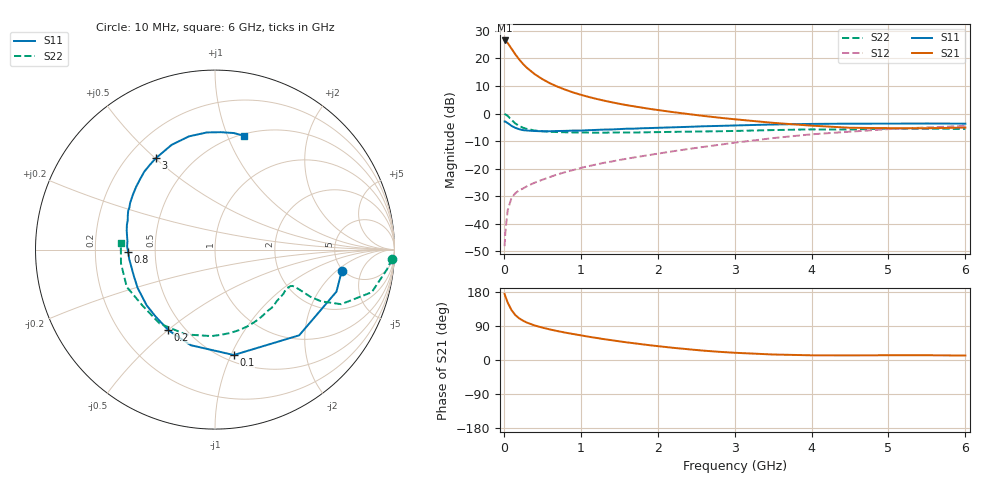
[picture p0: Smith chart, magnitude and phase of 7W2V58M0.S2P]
! Infineon Technologies  Discrete & RF Semiconductors
! BFS17W
! Si NPN RF Bipolar Junction Transistor in SOT323
! VCE = 2.5 V  IC = 8 mA
! Common Emitter S-Parameters:  August  1999
# GHz  S  MA  R  50
!  f  S11  S21  S12  S22
! GHz  MAG  ANG  MAG  ANG  MAG  ANG  MAG  ANG
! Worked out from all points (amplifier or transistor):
!   36 points, 10 MHz to 6 GHz, reference 50 ohm
!   highest |S21| = 26.5 dB at 10 MHz (marker M1)
!   |S21| within 3 dB of that: start of sweep to 100.4 MHz
!   unconditionally stable (mu >= 1): 434.1 MHz to 2.844 GHz; 4.192 GHz to end of sweep
!   at 250 MHz: K = 0.75, MSG = 22.6 dB, |S12| = -27.2 dB
!   at 1.4 GHz: K = 1.24, MAG = 7.8 dB, |S12| = -17.5 dB
!   at 6 GHz: K = 1.08, MAG = -2.0 dB, |S12| = -4.5 dB
!   S11 on the Smith chart (normalised r, x): 10 MHz: 4.84, -2.37; 100 MHz: 0.56, -1.02; 200 MHz: 0.41, -0.50; 800 MHz: 0.35, -0.01; 3 GHz: 0.31, +0.50; 6 GHz: 0.52, +1.15
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0.01  0.7161 -9.6  21.2 174.4  0.0039 85.6  0.9883 -2.9
0.02  0.7161 -19.1  20.9 168.0  0.007 81.2  0.9643 -6.6
0.05  0.6694 -45.5  19.09 151.5  0.0176 69.8  0.9052 -15.2
0.1  0.5965 -79.9  15.04 131.6  0.0293 58.4  0.7659 -23.4
0.15  0.5496 -104.3  11.82 118.4  0.0358 53.0  0.658 -26.0
0.2  0.5186 -120.1  9.556 109.9  0.0403 50.6  0.5935 -26.3
0.25  0.4984 -131.8  7.933 103.6  0.0435 50.5  0.5505 -25.8
0.3  0.4913 -140.8  6.758 98.7  0.0478 51.7  0.5249 -25.4
0.4  0.4811 -153.5  5.201 91.2  0.0554 53.8  0.4918 -25.0
0.5  0.4756 -162.0  4.215 85.5  0.0626 56.1  0.4771 -25.1
0.6  0.476 -168.5  3.536 80.6  0.0703 58.1  0.4663 -25.9
0.7  0.481 -173.8  3.063 76.2  0.0787 59.9  0.46 -27.3
0.8  0.4838 -178.4  2.701 72.2  0.0862 60.9  0.4559 -29.0
1.1  0.4975 170.4  2.004 61.5  0.1106 63.1  0.451 -35.4
1.3  0.5102 164.1  1.717 55.1  0.1272 63.9  0.4485 -40.6
1.6  0.5298 155.9  1.416 46.5  0.1511 64.7  0.4504 -48.6
2.2  0.5613 141.6  1.06 32.2  0.2063 65.5  0.4643 -66.8
3  0.6064 123.0  0.786 19.1  0.295 62.3  0.4823 -92.3
3.5  0.6317 112.5  0.677 14.5  0.3579 58.1  0.5001 -109.1
4.5  0.6543 94.0  0.551 12.1  0.4675 45.8  0.5107 -142.9
5.5  0.6578 80.9  0.54 12.6  0.5588 33.6  0.5294 -171.6
6  0.6545 75.8  0.555 11.7  0.5952 27.6  0.5264 175.8
